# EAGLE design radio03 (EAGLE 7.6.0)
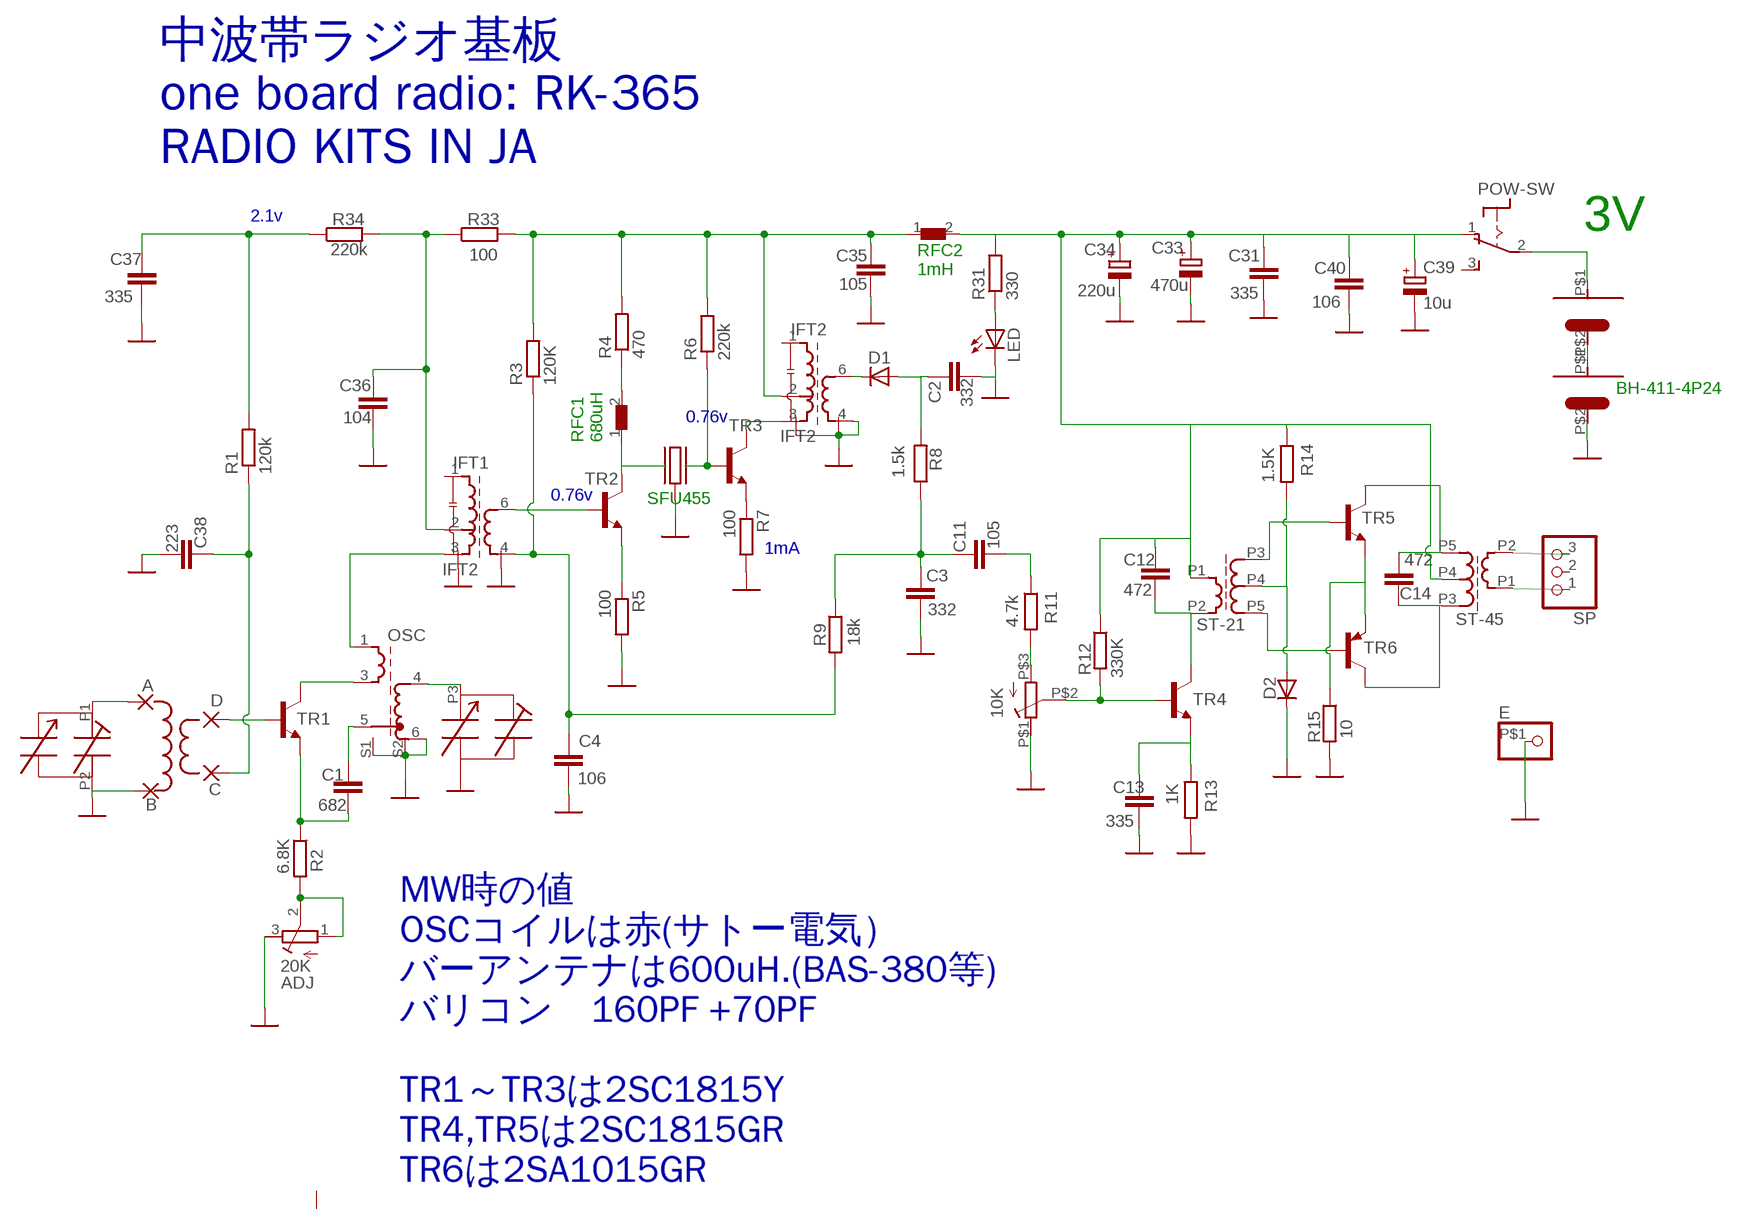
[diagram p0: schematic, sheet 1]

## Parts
10K  SINGLE-VR  [SINGLE-VR]
A  2,15/1,0  [2,15/1,0]
ADJ  20K  R-TRIMM3296W  [RTRIM3296W]
B  2,15/1,0  [2,15/1,0]
C  2,15/1,0  [2,15/1,0]
C1  682  C-EU050-024X044  [C050-024X044]
C2  332  C-EU050-024X044  [C050-024X044]
C3  332  C-EU050-024X044  [C050-024X044]
C4  106  C-EU050-024X044  [C050-024X044]
C11  105  C-EU050-024X044  [C050-024X044]
C12  472  C-EU050-024X044  [C050-024X044]
C13  335  C-EU050-024X044  [C050-024X044]
C14  472  C-EU050-024X044  [C050-024X044]
C31  335  C-EU050-024X044  [C050-024X044]
C33  470u  CPOL-EUE2.5-7  [E2,5-7]
C34  220u  CPOL-EUE2.5-6  [E2,5-6]
C35  105  C-EU050-024X044  [C050-024X044]
C36  104  C-EU050-024X044  [C050-024X044]
C37  335  C-EU050-024X044  [C050-024X044]
C38  223  C-EU050-024X044  [C050-024X044]
C39  10u  CPOL-EUE2.5-7  [E2,5-7]
C40  106  C-EU050-024X044  [C050-024X044]
D  2,15/1,0  [2,15/1,0]
D1  DIODE-D-5  [D-5]
D2  DIODE-D-5  [D-5]
E  PINHD-1X1  [1X01]
IFT1  IFT2  [FCZ]
IFT2  IFT2  [FCZ]
LED  LEDIRL80A  [IRL80A]
OSC  OSC-RED  [OSC-RED]
R1  120k  R-EU_0204/5  [0204/5]
R2  6.8K  R-EU_0204/5  [0204/5]
R3  120K  R-EU_0204/5  [0204/5]
R4  470  R-EU_0204/5  [0204/5]
R5  100  R-EU_0204/5  [0204/5]
R6  220k  R-EU_0204/5  [0204/5]
R7  100  R-EU_0204/5  [0204/5]
R8  1.5k  R-EU_0204/5  [0204/5]
R9  18k  R-EU_0204/5  [0204/5]
R11  4.7k  R-EU_0204/5  [0204/5]
R12  330K  R-EU_0204/5  [0204/5]
R13  1K  R-EU_0204/5  [0204/5]
R14  1.5K  R-EU_0204/5  [0204/5]
R15  10  R-EU_0204/5  [0204/5]
R31  330  R-EU_0204/5  [0204/5]
R33  100  R-EU_0204/5  [0204/5]
R34  220k  R-EU_0204/5  [0204/5]
RFC1  8101  [8101]
RFC2  8101  [8101]
SFU  SFU455  [SFU455]
SP  PINHD-1X3  [1X03]
ST-21  ST-32  [ST-32]
ST-45  ST-32  [ST-32]
TR1  2SC1815L  [TO92-1815]
TR2  2SC1815L  [TO92-1815]
TR3  2SC1815L  [TO92-1815]
TR4  2SC1815L  [TO92-1815]
TR5  2SC1815L  [TO92-1815]
TR6  2SA1015  [TO92-BCE]
U$2  VARI-C2  [VARI-C2]
U$3  BATTERY-AAA  [BATTERY-AAA]
U$4  BATTERY-AAA  [BATTERY-AAA]
U$5  POW-SW  [POW-SW]

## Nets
5V1: C12.2 C31.2 C33.+ C34.+ C39.+ C40.1 R12.1 R14.1 R31.2 RFC2.2 ST-21.P1 ST-45.P4 U$5.1(O)
GND: 10K.P$1(A) ADJ.3(A) B.1(P) C2.2 C3.2 C4.2 C13.1 C31.1 C33.- C34.- C35.2 C36.2 C37.2 C38.2 C39.- C40.2 D2.C E.P$1 IFT1.S1 IFT1.S2 IFT2.4 IFT2.S1 IFT2.S2 LED.K(C) OSC.6 OSC.S1 OSC.S2 R5.2 R7.2 R13.2 R15.2 SFU.2(G) U$2.P2(PCENTER) U$4.P$2
N$1: IFT2.3 TR3.C
N$3: C13.2 R13.1 TR4.E
N$4: D.1(P) TR1.B
N$5: 10K.P$3(E) R11.2
N$6: C12.1 ST-21.P2 TR4.C
N$7: U$3.P$2 U$4.P$1
N$8: ST-21.P3 TR5.B
N$9: R15.1 TR5.E TR6.E
N$10: U$3.P$1 U$5.2(P)
N$11: C3.1 C11.1 R8.1 R9.1
N$12: ST-21.P5 TR6.B
N$13: D2.A R14.2 ST-21.P4
N$14: C14.2 ST-45.P3 TR6.C
N$15: C14.1 ST-45.P5 TR5.C
N$16: SP.1 ST-45.P1
N$17: 10K.P$2(S) R12.2 TR4.B
N$18: SP.3 ST-45.P2
N$19: C11.2 R11.1
N$20: C2.1 D1.A R8.2
N$22: A.1(P) U$2.P1
N$23: C1.1 OSC.5
N$24: C1.2 R2.1 TR1.E
N$25: OSC.4 U$2.P3
N$26: C38.1 C.1(P) R1.1
N$27: IFT1.6 TR2.B
N$28: C4.1 IFT1.4 R3.1 R9.2
N$30: R5.1 TR2.E
N$31: C36.1 IFT1.2 R33.1 R34.2
N$32: C35.1 IFT2.2 R3.2 R4.2 R6.2 R33.2 RFC2.1
N$35: R6.1 SFU.3(OUT) TR3.B
N$36: RFC1.1 SFU.1(IN) TR2.C
N$37: R4.1 RFC1.2
N$39: R7.1 TR3.E
N$40: D1.C IFT2.6
N$47: C37.1 R1.2 R34.1
N$48: OSC.3 TR1.C
N$49: IFT1.3 OSC.1
N$50: ADJ.1(E) ADJ.2(S) R2.2
N$63: LED.A R31.1
Unconnected: IFT1.1 IFT2.1 SP.2 U$5.3(S)

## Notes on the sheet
- 中波帯ラジオ基板
  one board radio: RK-365
  RADIO KITS IN JA
- 2.1v
- 3V
- RFC2
  1mH
- BH-411-4P24
- 0.76v
- RFC1
  680uH
- 0.76v | SFU455
- 1mA
- MW時の値
  OSCコイルは赤(サトー電気）
  バーアンテナは600uH.(BAS-380等)
  バリコン　160PF +70PF
  
  TR1～TR3は2SC1815Y
  TR4,TR5は2SC1815GR
  TR6は2SA1015GR

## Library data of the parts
10K = resistor:SINGLE-VR
A B C D = wirepad:2,15/1,0: THROUGH-HOLE PAD
ADJ = resistor:R-TRIMM: Trimm resistor
C1-C4 C11-C14 C31 C35-C38 C40 = resistor:C-EU: CAPACITOR, European symbol
C33 C34 C39 = resistor:CPOL-EU: POLARIZED CAPACITOR, European symbol
D1 D2 = diode:DIODE-: DIODE
E = pinhead:PINHD-1X1: PIN HEADER
IFT1 IFT2 = OSC:IFT2
LED = led:LED: LED
OSC = OSC:OSC-RED
R1-R9 R11-R15 R31 R33 R34 = resistor:R-EU_: RESISTOR, European symbol
RFC1 RFC2 = inductors:8101
SFU = OSC:SFU455
SP = pinhead:PINHD-1X3: PIN HEADER
ST-21 ST-45 = OSC:ST-32
TR1-TR5 = transistor:2SC1815L
TR6 = transistor-pnp:2SA1015
U$2 = OSC:VARI-C2
U$3 U$4 = OSC:BATTERY-AAA
U$5 = switch:POW-SW

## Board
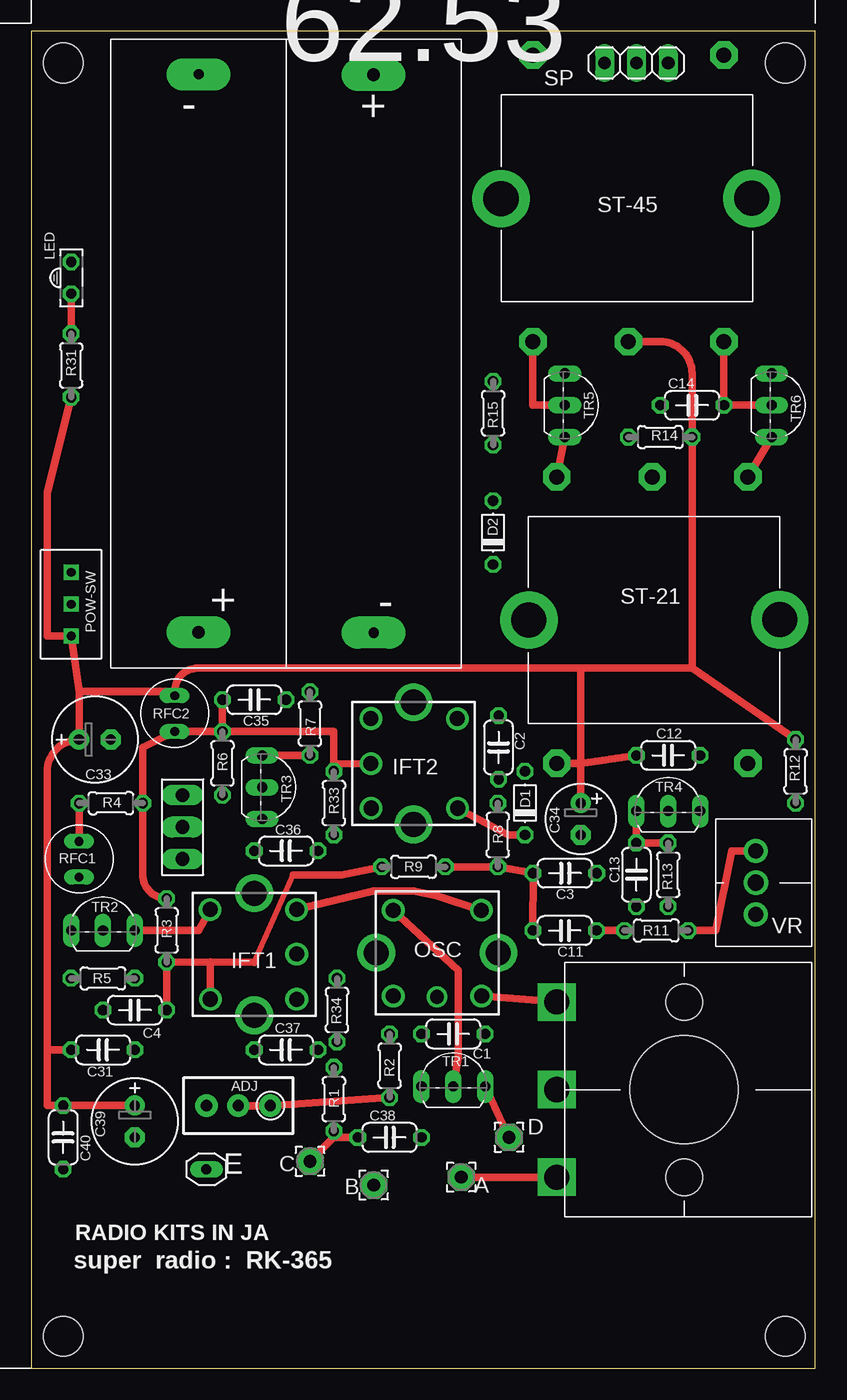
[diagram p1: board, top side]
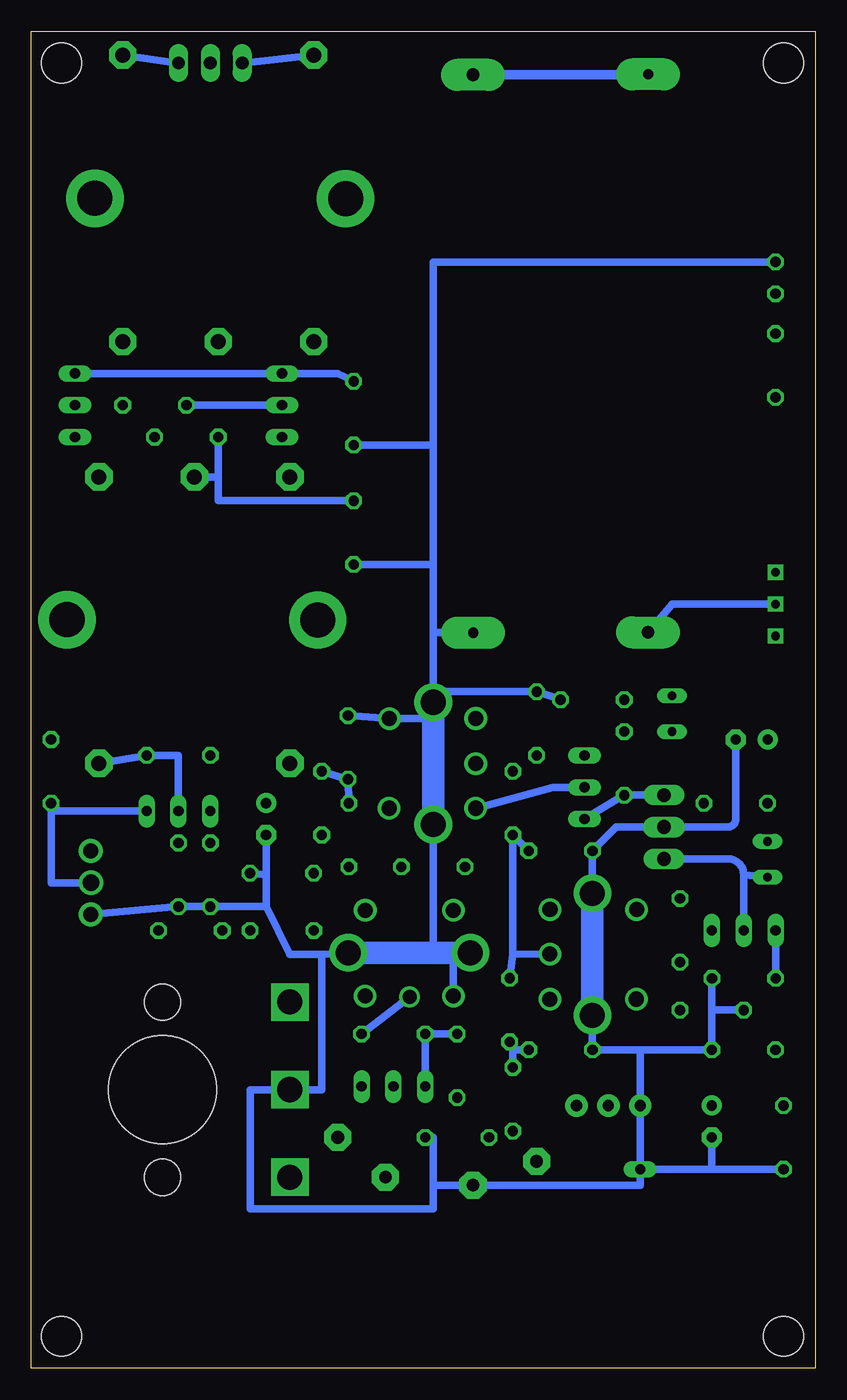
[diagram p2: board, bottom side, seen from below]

Size 62.53 x 106.67 mm. Coordinates in mm from the lower left corner, seen from the top.
Outline: 0,0 62.53,0 62.53,106.67 0,106.67 0,0
Copper layers (1*16): Top 0.035mm / dielectric 1.5mm / Bottom 0.035mm
Design rules "default": minimum track width 10mil, minimum drill 24mil, track to track 8mil, track to pad 8mil, pad to pad 8mil, via to via 8mil, smd to smd 8mil, copper to edge 40mil, drill to drill 8mil, minimum pad ring 10mil, minimum via ring 8mil, stop-mask expansion 4mil, vias tented up to drill 0mil, thermal gap 10mil
Holes 3.2 mm at 2.54,2.54 60.13,2.54 2.54,104.14 60.13,104.14

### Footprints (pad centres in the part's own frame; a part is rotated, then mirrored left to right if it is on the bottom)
SINGLE-VR = drill 1.2 pad 1.93: P$1 0.635,2.54; P$3 0.635,-2.54 | drill 1.3 pad 1.93: P$2 0.635,0
2,15/1,0 = drill 1.016 pad 2.159 octagon: 1 0,0
RTRIM3296W = drill 0.9 pad 1.778: 1 0,-2.54; 2 0,0; 3 0,2.54
C050-024X044 = drill 0.813 octagon: 1 -2.54,0; 2 2.54,0
E2,5-7 = drill 0.813 pad 1.6: + -1.27,0 | drill 0.813 pad 1.6 octagon: - 1.27,0
E2,5-6 = drill 0.813 pad 1.6: + -1.27,0 | drill 0.813 pad 1.6 octagon: - 1.27,0
D-5 = drill 0.813 octagon: A 2.54,0; C -2.54,0
1X01 = drill 0.8 long: P$1 0,0
FCZ = drill 1.2: 1 -3.39,3.581; 2 -3.39,-0.025; 3 -3.384,-3.581; 4 3.498,3.575; 6 3.518,-3.581 | drill 2: S1 0,-4.873; S2 0,4.873
IRL80A = drill 0.813 octagon: A 0,-1.27; K 0,1.27
OSC-RED = drill 1.2: 1 -3.39,3.518; 3 -3.39,-3.518; 4 3.454,3.531; 6 3.454,-3.518 | drill 1.1: 5 3.518,-0.025 | drill 2: S1 0,-4.873; S2 0,4.873
0204/5 = drill 0.813 octagon: 1 -2.54,0; 2 2.54,0
8101 = drill 0.7 pad 0.813 long: 1 0,1.46; 2 0,-1.397
SFU455 = drill 1.1 long: 1 -2.54,0; 3 2.54,0 | drill 1.1 pad 1.676 long: 2 0,0
1X03 = drill 1.016 long: 1 -2.54,0; 2 0,0; 3 2.54,0
ST-32 = drill 1.2 pad 2.184 octagon: P1 -11.43,7.62; P2 -11.43,-7.62; P3 11.43,7.62; P4 11.43,0; P5 11.43,-7.62 | drill 2.8 pad 4.572: P$1 0,9.842; P$2 0.032,-10.16
TO92-1815 = drill 0.813 long: B 2.54,0; C 0,0; E -2.54,0
TO92-BCE = drill 0.813 long: B 2.54,0; C 0,0; E -2.54,0
VARI-C2 = drill 2 square: P1 10.16,6.985; P2 10.16,0; P3 10.16,-6.985 | hole 2.921: 0,6.985; 0,-6.985 | hole 8.636: 0,0
BATTERY-AAA = drill 1 pad 2.54 long: P$1 2.838,0 | drill 0.8 pad 2.54 long: P$2 47.365,0
POW-SW = drill 0.7 square: 1 -3.81,0; 2 -1.27,0; 3 1.27,0

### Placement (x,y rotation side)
10K  58.42,38.73 180 top
A  34.29,15.24 0 top
ADJ  16.51,20.95 90 top
B  27.3,14.61 0 top
C  22.23,16.51 0 top
C1  33.66,26.67 180 top
C2  37.27,49.53 90 top
C3  42.56,39.5 0 top
C4  8.26,28.57 180 top
C11  42.55,34.92 0 top
C12  50.8,48.9 180 top
C13  48.26,39.37 90 top
C14  52.7,76.83 0 top
C31  5.71,25.4 180 top
C33  5.07,50.15 0 top
C34  43.81,43.81 270 top
C35  17.78,53.34 0 top
C36  20.32,41.27 180 top
C37  20.32,25.4 180 top
C38  28.57,18.41 0 top
C39  8.26,19.68 270 top
C40  2.54,18.41 270 top
D  38.1,18.41 0 top
D1  39.37,45.09 90 top
D2  36.83,66.67 90 top
E  13.97,15.88 180 top
IFT1  17.78,33.02 180 top
IFT2  30.48,48.26 0 top
LED  3.17,87 0 top
OSC  32.38,33.15 270 top
R1  24.13,21.46 90 top
R2  28.57,24.13 270 top
R3  10.79,34.93 90 top
R4  6.35,45.09 0 top
R5  5.71,31.11 0 top
R6  15.24,48.26 90 top
R7  22.23,51.44 90 top
R8  37.21,42.55 90 top
R9  30.48,40.01 180 top
R11  49.85,34.92 0 top
R12  60.96,47.62 270 top
R13  50.8,39.37 270 top
R14  50.16,74.3 180 top
R15  36.83,76.2 270 top
R31  3.17,80.01 270 top
R33  24.13,45.09 90 top
R34  24.38,28.57 90 top
RFC1  3.81,40.64 180 top
RFC2  11.43,52.26 180 top
SFU  12.06,43.18 90 top
SP  48.26,104.14 180 top
ST-21  49.53,59.69 90 top
ST-45  47.62,93.34 270 top
TR1  33.66,22.48 0 top
TR2  5.71,34.93 0 top
TR3  18.41,46.35 270 top
TR4  50.8,44.45 0 top
TR5  42.55,76.83 270 top
TR6  59.05,76.83 270 top
U$2  52.07,22.23 180 top
U$3  13.34,55.88 90 top
U$4  27.3,106.05 270 top
U$5  3.17,62.23 90 top

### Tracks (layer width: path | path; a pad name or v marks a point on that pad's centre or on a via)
5V1
  Top 0.61: 43.81,48.26 C12.2 | 52.7,55.88 R14.1 52.7,79.38 arc90 50.16,81.92 ST-45.P4 | C34.+ 43.81,48.26 | R12.1 52.7,55.88 | 52.7,55.88 43.81,55.88 | 43.81,55.88 13.34,55.88 arc90 11.43,53.98 | 43.81,48.26 43.81,55.88 | ST-21.P1 43.81,48.26 | 1.27,25.4 1.27,47.62 arc-90 C33.+ 3.81,53.98 | C31.2 1.27,25.4 | 3.81,53.98 U$5.1 1.27,58.42 1.27,69.85 R31.2 | 3.81,53.98 11.43,53.98 | 11.43,53.98 arc90 11.3,53.85 RFC2.2 | 1.27,25.4 1.27,20.95 C40.1 C39.+
GND
  Bottom 0.61: 30.49,51.85 IFT2.4 C2.2 | IFT1.S1 C36.2 15.88,43.18 SFU.2 6.99,43.18 arc-90 6.35,43.81 6.35,47.62 C33.- | IFT1.S2 C37.2 13.97,25.4 | 10K.P$1 R13.2 C13.1 43.81,36.83 | 30.48,53.98 IFT2.S2 30.48,53.98 | OSC.6 28.89,33.15 | IFT2.S1 30.48,33.15 | 13.96,23.5 arc-90 13.97,23.5 | E.P$1 ADJ.3 13.97,23.5 | E.P$1 13.97,14.61 B.1 30.48,14.61 | OSC.S2 39.37,33.02 | 39.37,33.02 39.37,22.23 U$2.P2 45.09,22.23 45.09,12.7 30.48,12.7 30.48,14.61 | 39.37,33.02 41.91,33.02 43.81,36.83 | D2.C 30.48,64.14 | 30.48,64.14 30.47,58.7 | 30.47,58.7 30.48,53.98 | U$4.P$2 30.47,58.7 | C34.- 43.81,39.37 | 43.81,39.37 43.81,36.83 | C3.2 43.81,39.37 | C40.2 8.26,15.88 | 8.26,15.88 E.P$1 | C39.- 8.26,15.88 | 13.97,25.4 C31.1 8.25,28.58 | LED.K 30.48,88.27 30.48,73.66 | 30.48,73.66 30.48,64.14 | R15.2 30.48,73.66 | 30.48,53.98 R7.2 C35.2 | R5.2 8.25,28.58 | C4.2 8.25,28.58 | 13.97,25.4 13.97,23.5 | C38.2 30.48,18.41 30.48,14.61
  Bottom 1.778: IFT2.S2 30.49,51.85 IFT2.S1 | IFT1.S1 IFT1.S2 | OSC.S2 30.48,33.15 28.89,33.15 OSC.S1
N$1
  Bottom 0.61: TR3.C 20.95,46.35 IFT2.3
N$3
  Top 0.61: TR4.E C13.2 R13.1
N$4
  Top 0.61: TR1.B D.1
N$5
  Top 0.61: R11.2 54.61,34.92 55.88,41.27 10K.P$3
N$6
  Bottom 0.61: ST-21.P2 C12.1 50.8,48.9 TR4.C
N$7
  Bottom 0.813: U$4.P$1 U$3.P$2
N$8
  Top 0.61: ST-21.P3 TR5.B
N$9
  Bottom 0.61: TR6.E TR5.E 38.1,79.38 R15.1
N$10
  Bottom 0.61: U$5.2 11.43,60.96 U$3.P$1
N$11
  Top 0.61: R9.1 R8.1 C3.1 C11.1
N$12
  Top 0.61: TR6.B ST-21.P5
N$13
  Bottom 0.61: D2.A 47.62,69.22 47.62,71.12 | 47.62,71.12 R14.2 | ST-21.P4 47.62,71.12
N$14
  Top 0.61: ST-45.P3 C14.2 TR6.C
N$15
  Top 0.61: ST-45.P5 40.01,76.83 TR5.C
  Bottom 0.61: C14.1 TR5.C
N$16
  Bottom 0.61: ST-45.P1 SP.1
N$17
  Bottom 0.61: R12.2 60.96,44.45 | 60.96,44.45 TR4.B | 10K.P$2 60.96,38.73 60.96,44.45
N$18
  Bottom 0.61: ST-45.P2 SP.3
N$19
  Top 0.61: C11.2 R11.1
N$20
  Bottom 0.61: D1.A C2.1 R8.2
N$22
  Top 0.61: A.1 U$2.P1
N$23
  Bottom 0.61: OSC.5 C1.1
N$24
  Bottom 0.61: R2.1 C1.2 TR1.E
N$25
  Top 0.61: OSC.4 U$2.P3
N$26
  Top 0.61: R1.1 24.13,18.41 | 24.13,18.41 C.1 | C38.1 24.13,18.41
N$27
  Top 0.61: IFT1.6 13.34,34.92 TR2.B
N$28
  Top 0.406: 17.79,32.39 20.87,39.37
  Top 0.61: 20.87,39.37 24.77,39.37 R9.2 | C4.1 R3.1 | R3.1 14.28,32.4 | R3.1 | 14.28,32.4 IFT1.4 | 14.28,32.4 17.79,32.39
N$30
  Bottom 0.61: TR2.E R5.1
N$31
  Bottom 0.61: 24.13,33.02 IFT1.2 | C36.1 R33.1 24.13,33.02 | 24.13,33.02 R34.2
N$32
  Top 0.61: R3.2 arc-90 8.89,39.38 R4.2 8.89,49.53 RFC2.1 R6.2 | R6.2 24.12,50.8 24.13,48.23 | 24.13,48.23 R33.2 | IFT2.2 24.13,48.23 | C35.1 R6.2
N$35
  Bottom 0.61: SFU.3 R6.1 TR3.B
N$36
  Bottom 0.61: SFU.1 6.99,40.64 arc90 5.71,39.37 | 5.71,39.37 TR2.C | RFC1.1 5.71,39.37
N$37
  Top 0.61: R4.1 RFC1.2
N$39
  Top 0.61: R7.1 TR3.E
N$40
  Top 0.61: IFT2.6 38.04,42.55 D1.C
N$47
  Bottom 0.61: C37.1 24.13,25.4 | 24.13,25.4 R1.2 | R34.1 24.13,25.4
N$48
  Top 0.61: OSC.3 34.04,31.75 34.04,24.77 TR1.C
N$49
  Top 0.61: OSC.1 32.38,37.68 30.48,38.1 27.3,38.1 IFT1.3
N$50
  Top 0.61: ADJ.2 ADJ.1 R2.2
N$63
  Top 0.61: R31.1 LED.A

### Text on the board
tNames: - | + | ST-45 | ST-21 | + | - | VR | RADIO KITS IN JA | super radio : RK-365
